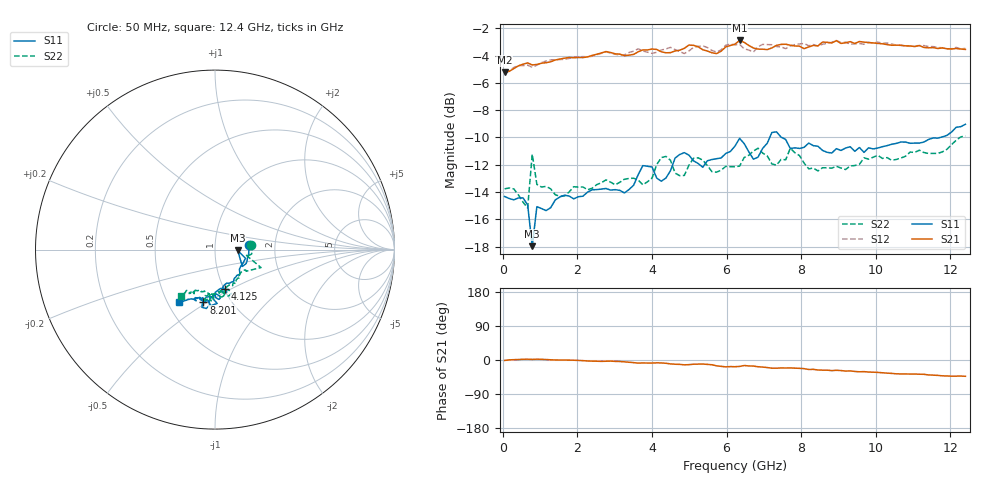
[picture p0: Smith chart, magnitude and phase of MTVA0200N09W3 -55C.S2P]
! Network Analyzer HP8720D.06.14 Serial No. US36140669
! 24 Jul 2008  11:07:52
! Frequency  S11  S21  S12  S22
# HZ  S  DB R 50
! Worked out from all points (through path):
!   101 points, 50 MHz to 12.4 GHz, reference 50 ohm
!   highest |S21| = -2.90 dB at 6.348 GHz (marker M1); lowest = -5.2 dB at 50 MHz (marker M2)
!   group delay of S21, straight-line fit = 10.8 ps
!   lowest |S11| = -18.0 dB at 791 MHz (marker M3), VSWR 1.29, Z = 64.5 - j0.634 ohm
!   |S11| at or under -10 dB: start of sweep to 7.156 GHz; 7.477 GHz to 11.73 GHz (4.25 GHz wide, 44.3 % of centre)
!   |S22| runs from -15.2 to -9.9 dB; largest |S21 - S12| = 0.038
!   S11 on the Smith chart (normalised r, x): 50 MHz: 1.47, +0.07; 4.125 GHz: 1.01, -0.46; 8.201 GHz: 0.75, -0.48; 12.4 GHz: 0.57, -0.38
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5e7  -14.32 7.2  -5.23 -1.2  -5.26 -0.9  -13.76 7.7
6.675e8  -14.94 -31.6  -4.54 2.2  -4.71 2.4  -15.17 -9.7
7.91e8  -17.96 -2.2  -4.69 1.5  -4.86 1.0  -11.22 -21.3
9.145e8  -15.07 -15.9  -4.66 2.2  -4.71 1.2  -13.44 -34.3
1.532e9  -14.36 -43.7  -4.26 -0.0  -4.30 0.4  -14.31 -40.2
2.1495e9  -14.30 -55.9  -4.15 -1.7  -4.08 -1.4  -13.62 -49.3
3.261e9  -14.06 -70.9  -4.01 -4.9  -3.95 -6.1  -13.06 -63.6
3.755e9  -12.06 -78.2  -3.59 -7.7  -3.67 -5.7  -13.47 -68.5
4.1255e9  -12.97 -75.4  -3.55 -7.5  -3.77 -9.3  -11.99 -78.7
4.249e9  -13.20 -81.6  -3.72 -7.7  -3.60 -9.7  -11.48 -74.8
4.743e9  -11.25 -87.1  -3.61 -11.6  -3.71 -9.7  -12.80 -76.7
5.3605e9  -12.18 -89.0  -3.57 -10.7  -3.29 -12.0  -11.66 -79.0
5.731e9  -11.56 -93.0  -3.86 -15.4  -3.74 -14.7  -12.54 -85.9
6.225e9  -10.63 -96.4  -3.17 -17.7  -3.22 -15.7  -12.14 -91.2
6.3485e9  -10.06 -94.6  -2.90 -17.0  -3.18 -15.3  -12.10 -94.4
6.719e9  -11.59 -93.2  -3.45 -16.0  -3.75 -18.7  -10.99 -96.0
7.213e9  -9.64 -102.8  -3.45 -21.6  -3.21 -19.2  -11.93 -92.9
7.707e9  -10.81 -96.9  -3.25 -20.9  -3.31 -23.3  -10.79 -101.2
8.201e9  -10.41 -102.3  -3.37 -25.1  -3.29 -23.3  -12.30 -100.4
8.3245e9  -10.60 -101.6  -3.26 -24.7  -3.20 -24.0  -12.24 -101.5
1.0424e10  -10.50 -112.0  -3.25 -35.3  -3.16 -35.3  -11.67 -117.5
1.24e10  -9.04 -124.3  -3.55 -43.0  -3.47 -42.7  -9.88 -126.2
